(* Logix 5000 AddOnInstructionDefinition export AMCI_5034_PTO_AM_Prog_Min_Reg_Dist; software revision 37.00 *)

TYPE AMCI_5034_PTO_AM_Input_Data :
STRUCT
   ConnectionFaulted : DINT;
   MovingCW : BOOL;
   MovingCCW : BOOL;
   InHoldState : BOOL;
   Stopped : BOOL;
   AtHome : BOOL;
   Accelerating : BOOL;
   Decelerating : BOOL;
   MoveComplete : BOOL;
   HomeInvalid : BOOL;
   InvalidProfile : BOOL;
   PositionInvalid : BOOL;
   InputError : BOOL;
   CommandError : BOOL;
   ConfigurationError : BOOL;
   ModuleOK : BOOL;
   GeneralPurposeOutputStatus : BOOL;
   Input1Active : BOOL;
   Input2Active : BOOL;
   Input3Active : BOOL;
   Input4Active : BOOL;
   bit_20_reserved : BOOL;
   bit_21_reserved : BOOL;
   bit_22_reserved : BOOL;
   EncoderFollowerMode : BOOL;
   BlendMoveRunning : BOOL;
   BlendMoveAcknowledge : BOOL;
   MinimumRegistrationProgrammed : BOOL;
   EncoderMotionDirection : BOOL;
   MultipleInputsWithSameFunction : BOOL;
   FSCExceedsNumberOfDataBits : BOOL;
   AbsoluteEncoderSetupError : BOOL;
   bit_31_reserved : BOOL;
   CurrentPosition : DINT;
   EncoderPosition : DINT;
   CapturedPosition : DINT;
END_STRUCT
END_TYPE

TYPE AMCI_5034_PTO_AM_Output_Data :
STRUCT
   Command_Word : DINT;
   TargetPosition : DINT;
   TargetVelocity : UDINT;
   Acceleration : DINT;
   Deceleration : DINT;
END_STRUCT
END_TYPE

ADD_ON_INSTRUCTION AMCI_5034_PTO_AM_Prog_Min_Reg_Dist   (* revision 1.0, vendor AMCI, ExecuteEnableInFalse *)
// AMCI Program Minimum Registration Distance
// Revision note:
// 10/01/2025 Intial release
// Help:
// AXIS INPUT DATA:  Input data from the AMCI 5034-PTO-AM.   Uses the AMCI_5034_PTO_Input_Data User Defined Data Type.
// AXIS OUTPUT DATA; Output data from the AOI to the AMCI 5034-PTO-AM.    Uses the AMCI_5034_PTO_Output_Data User Defined Data Type.
// TARGETPOSITION: The number of steps that must be output by the PTO module before it will start looking for the registration input.
// EN (Enable) Set when rung is true, Reset when rung is false
// DN (Done) Set when command is sent to the PTO module.  Reset when the rung is false.
// ER (Error) Set when a command, input error, or configuation error.   Reset when the rung is false.
VAR_IN_OUT
   Axis_Input_Data : AMCI_5034_PTO_AM_Input_Data; {required}
   Axis_Output_Data : AMCI_5034_PTO_AM_Output_Data; {required}
END_VAR
VAR_INPUT
   Minimum_Registration_Distance : DINT; {required}
END_VAR
VAR_OUTPUT
   EN : BOOL; {visible}   // set when rung with AOI is true
   DN : BOOL; {access Read Only, visible}   // set when mnimum registration distance has been programmed
   ER : BOOL; {access Read Only, visible}   // set when input, command, or configuraiton error
END_VAR
VAR
   command_data_block : DINT[5];
        [0]   // Command Bits MSW
        [1]   // Target Position
        [2]   // Upper Target Position
        [3]   // Lower Target Position
        [4]   // Upper Programmed Speed
END_VAR

ROUTINE EnableInFalse   (* ladder *)
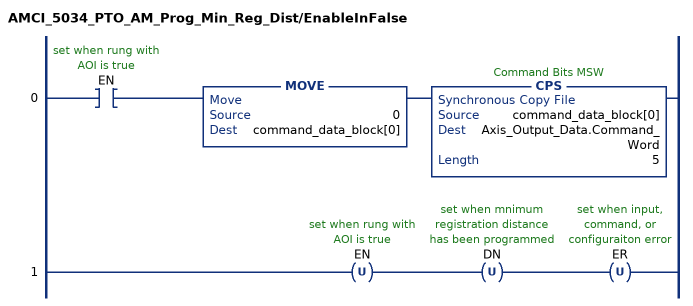
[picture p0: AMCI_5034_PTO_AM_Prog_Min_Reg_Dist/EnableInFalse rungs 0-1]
   0: XIC(EN)MOVE(0,command_data_block[0])CPS(command_data_block[0],Axis_Output_Data.Command_Word,5);
   1: OTU(EN)OTU(DN)OTU(ER);
END_ROUTINE

ROUTINE Logic   (* ladder *)
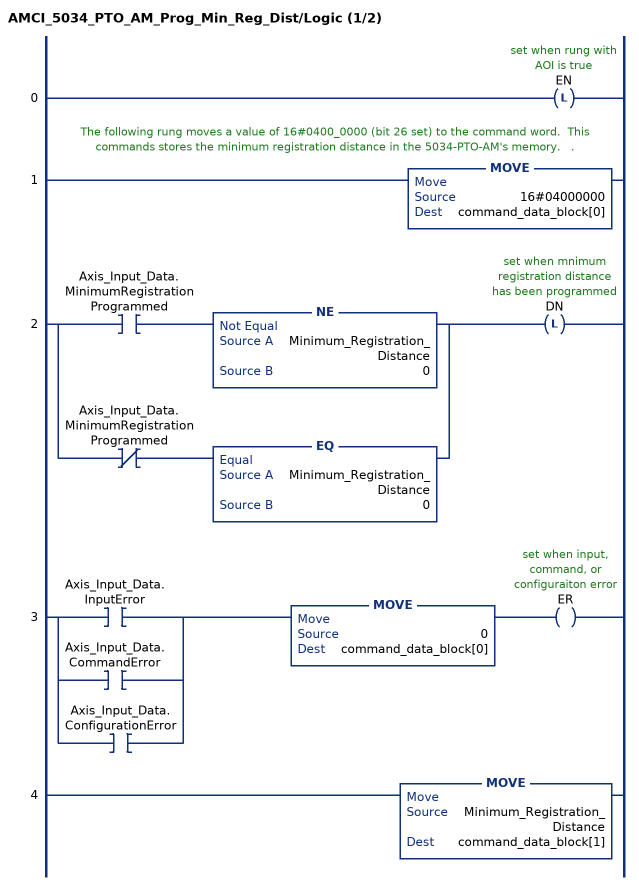
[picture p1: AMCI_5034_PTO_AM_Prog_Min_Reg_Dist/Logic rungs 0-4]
   0: OTL(EN);
   // The following rung moves a value of 16#0400_0000 (bit 26 set) to the command word.  This commands stores the minimum registration distance in the 5034-PTO-AM's memory.   .
   1: MOVE(16#04000000,command_data_block[0]);
   2: [XIC(Axis_Input_Data.MinimumRegistrationProgrammed) NE(Minimum_Registration_Distance,0) ,XIO(Axis_Input_Data.MinimumRegistrationProgrammed) EQ(Minimum_Registration_Distance,0) ]OTL(DN);
   3: [XIC(Axis_Input_Data.InputError) ,XIC(Axis_Input_Data.CommandError) ,XIC(Axis_Input_Data.ConfigurationError) ]MOVE(0,command_data_block[0])OTE(ER);
   4: MOVE(Minimum_Registration_Distance,command_data_block[1]);
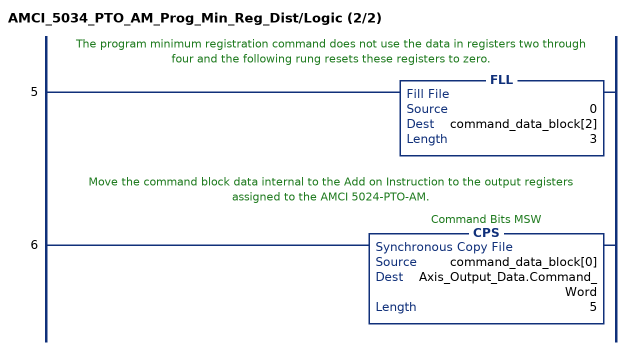
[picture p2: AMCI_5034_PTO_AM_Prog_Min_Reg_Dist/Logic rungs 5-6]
   // The program minimum registration command does not use the data in registers two through four and the following rung resets these registers to zero.
   5: FLL(0,command_data_block[2],3);
   // Move the command block data internal to the Add on Instruction to the output registers assigned to the AMCI 5024-PTO-AM.
   6: CPS(command_data_block[0],Axis_Output_Data.Command_Word,5);
END_ROUTINE
END_ADD_ON_INSTRUCTION
